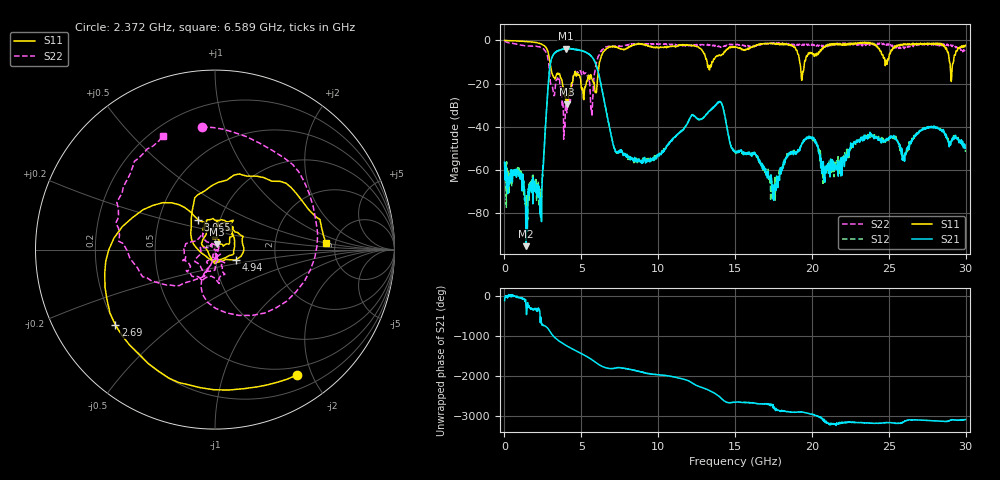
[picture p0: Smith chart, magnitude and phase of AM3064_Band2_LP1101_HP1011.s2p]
# Hz S DB R 50.0
!freq dBS11 angS11 dBS21 angS21 dBS12 angS12 dBS22 angS22
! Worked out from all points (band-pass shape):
!   1600 points, 10 MHz to 29.98 GHz, reference 50 ohm
!   highest |S21| = -3.79 dB at 4.002 GHz (marker M1); lowest = -95.3 dB at 1.397 GHz (marker M2)
!   |S21| within 3 dB of the highest: 3.165 GHz to 5.578 GHz (2.413 GHz wide, 55.2 % of centre)
!   lowest |S11| = -29.7 dB at 4.04 GHz (marker M3), VSWR 1.07, Z = 51.2 + j3.1 ohm
!   |S11| at or under -10 dB: 2.955 GHz to 6.188 GHz (3.233 GHz wide, 70.7 % of centre); 13.18 GHz to 13.5 GHz (319.3 MHz wide, 2.39 % of centre); 19.19 GHz to 19.52 GHz (325.4 MHz wide, 1.68 % of centre)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
!   |S22| runs from -45.8 to -0.3 dB; largest |S21 - S12| = 0.017
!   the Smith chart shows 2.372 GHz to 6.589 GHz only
!   S11 on the Smith chart (normalised r, x): 2.372 GHz: 0.39, -1.78; 2.69 GHz: 0.20, -0.32; 3.065 GHz: 0.79, +0.27; 4.94 GHz: 1.26, -0.14; 6.589 GHz: 4.20, +0.46
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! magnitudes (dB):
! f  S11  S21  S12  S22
! 10 MHz  0.0  -56.4  -56.6  -0.3
! 1.397 GHz  -0.5  -95.3  -71.9  -2.5
! 2.372 GHz  -1.6  -72.9  -82.1  -3.3
! 2.69 GHz  -3.1  -37.3  -37.1  -5.3
! 3.065 GHz  -14.3  -8.4  -8.3  -20.9
! 4.002 GHz  -27.0  -3.8  -3.8  -31.1
! 4.04 GHz  -29.7  -3.9  -3.9  -31.6
! 4.94 GHz  -17.6  -4.8  -4.7  -14.1
! 5.015 GHz  -22.2  -4.7  -4.7  -15.7
! 5.671 GHz  -17.6  -7.5  -7.5  -33.1
! 6.589 GHz  -4.2  -31.7  -31.4  -3.1
! 7.283 GHz  -3.3  -51.8  -52.2  -2.6
! 10 GHz  -3.4  -52.8  -52.6  -1.8
! 13.97 GHz  -6.7  -28.7  -28.4  -2.8
! 15 GHz  -2.9  -51.7  -52.0  -1.8
! 17.46 GHz  -1.3  -73.4  -70.7  -1.4
! 19.35 GHz  -17.8  -47.6  -47.9  -2.3
! 19.99 GHz  -5.7  -45.2  -45.2  -1.8
! 20.83 GHz  -3.2  -65.7  -60.8  -2.3
! 25 GHz  -8.3  -45.7  -45.2  -1.7
! 29.08 GHz  -17.8  -46.4  -46.3  -2.5
! 29.98 GHz  -2.3  -49.8  -51.6  -4.7
